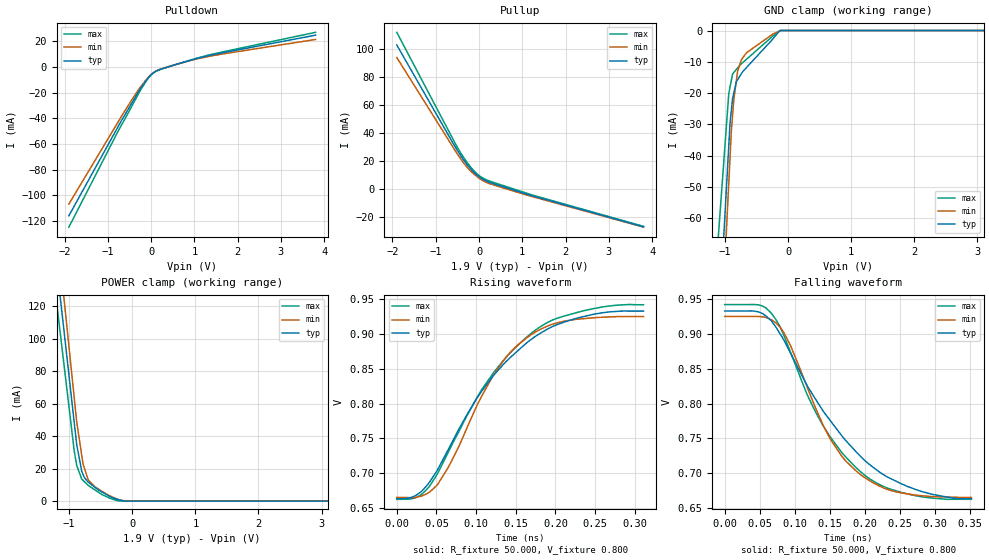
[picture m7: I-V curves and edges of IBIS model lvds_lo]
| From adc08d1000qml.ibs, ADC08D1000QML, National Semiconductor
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[Model]   lvds_lo
Model_type Output
Vref=8.000E-01
Rref=5.000E+01
Cref=2.500E-12
Vmeas=8.000E-01
C_comp   5.910E-13   5.910E-13   5.910E-13
[Voltage Range]   1.900E+00   1.800E+00   2.000E+00
[POWER Clamp Reference]   1.900E+00   1.800E+00   2.000E+00
[GND Clamp Reference]   0.000E+00   0.000E+00   0.000E+00
[Pullup Reference]   1.900E+00   1.800E+00   2.000E+00
[Pulldown Reference]   0.000E+00   0.000E+00   0.000E+00
[Temperature Range]   25   125   -55
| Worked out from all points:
|   slope of the pulldown table from 0 to 0.285 V, typ, clamps not added: 57.1 ohm
|   slope of the pullup table from 0 to 0.285 V, typ, clamps not added: 62.9 ohm
|   GND clamp passes 1 mA (typ) near -0.17 V on its own axis
|   POWER clamp passes 1 mA (typ) near -0.23 V on its own axis
|   rising waveform, R_fixture 50.000, V_fixture 0.800: 20-80 % time 98.3ps typ, 73.8ps min, 95ps max; typ from 0.664 V to 0.933 V
|   falling waveform, R_fixture 50.000, V_fixture 0.800: 20-80 % time 110ps typ, 74.9ps min, 88.3ps max; typ from 0.933 V to 0.664 V
[GND Clamp]
-2V       -423.4mA   -483.1mA   -312.6mA
-1.8V     -350.5mA   -401.2mA   -257.4mA
-940mV    -36.84mA   -48.8mA    -20.2mA
-920mV    -29.54mA   -40.6mA    -18.1mA
-900mV    -25.67mA   -32.41mA   -16mA
-860mV    -19.99mA   -22.06mA   -13.41mA
-800mV    -15.75mA   -13.08mA   -11.95mA
-740mV    -13.81mA   -9.307mA   -10.63mA
-660mV    -11.86mA   -7.124mA   -9.203mA
-240mV    -2.641mA   -1.106mA   -1.734mA
-130mV    0A         -92.15uA   -144.5uA
4V        0A         0A         0A
[Power Clamp]
-2.1V     459.4mA    508.4mA    418mA
-1.7V     320.1mA    357.7mA    286.8mA
-1V       76.45mA    94mA       57.24mA
-920mV    48.6mA     63.86mA    31mA
-880mV    34.67mA    48.79mA    21.92mA
-800mV    18.35mA    28.08mA    13.57mA
-780mV    16.52mA    22.91mA    12.8mA
-700mV    11.75mA    13.25mA    9.727mA
-480mV    5.631mA    6.059mA    4.013mA
-240mV    1.077mA    1.278mA    270.4uA
-120mV    0A         761.7pA    0A
3.9V      0A         0A         0A
[Pullup]
-1.9V     102.9mA    93.87mA    111.9mA
-480mV    26.44mA    23.87mA    28.54mA
-340mV    19.83mA    17.76mA    21.61mA
-200mV    14.37mA    12.81mA    15.72mA
20mV      8.132mA    7.106mA    8.969mA
240mV     4.574mA    3.628mA    5.512mA
1.18V     -4.688mA   -5.255mA   -4.034mA
3.8V      -27.31mA   -27.56mA   -26.98mA
[Pulldown]
-1.9V     -116mA     -106.9mA   -124.9mA
-700mV    -42.75mA   -39.39mA   -46.27mA
-260mV    -17.71mA   -16.35mA   -19.05mA
-60mV     -8.319mA   -7.995mA   -8.603mA
60mV      -4.48mA    -4.403mA   -4.564mA
160mV     -2.631mA   -2.531mA   -2.748mA
400mV     52.84uA    130.2uA    -30.36uA
1.3V      8.459mA    7.913mA    8.957mA
3.8V      24.69mA    21.33mA    26.89mA
[Rising Waveform]
R_fixture = 50.000
V_fixture = 0.800
V_fixture_min = 0.800
V_fixture_max = 0.800
|  time   V(typ)   V(min)   V(max)
0s        663.8mV    665.5mV    662.7mV
29.5ps    672.7mV    666.9mV    668.5mV
51.5ps    705.3mV    684mV      699.8mV
88.5ps    784mV      765.5mV    782.9mV
122ps     840.6mV    841.3mV    844.3mV
144ps     867.1mV    874.7mV    873.9mV
165.5ps   888.8mV    895.7mV    897.1mV
194.5ps   909.5mV    913.3mV    919mV
227.5ps   922.7mV    921mV      930.8mV
311ps     932.7mV    924.9mV    941.8mV
[Falling Waveform]
R_fixture = 50.000
V_fixture = 0.800
V_fixture_min = 0.800
V_fixture_max = 0.800
|  time   V(typ)   V(min)   V(max)
0s        932.7mV    924.9mV    941.8mV
53ps      929.3mV    924.4mV    940mV
78.5ps    900.8mV    910.1mV    911mV
94.5ps    871.2mV    881.9mV    872mV
116.5ps   827.8mV    827.1mV    815.5mV
139.5ps   790.6mV    771mV      769.7mV
166.5ps   754.6mV    725.3mV    730.5mV
201ps     717.3mV    693.1mV    696.2mV
271.5ps   677.1mV    668.7mV    668.1mV
352ps     663.8mV    665.5mV    662.7mV
[Ramp]
dV/dt_f   1.7617E+00/1.0991E-10   1.7025E+00/7.4484E-11   1.8218E+00/8.7898E-11
dV/dt_r   1.7617E+00/9.8080E-11   1.7025E+00/7.3700E-11   1.8218E+00/9.4780E-11
R_load = 50
